// TwinCAT 3 PLC project Plc01_TrafficLightSystem
// ProgramVersion: 3.1.4020.4
// libraries:
//   Tc2_Standard, * (Beckhoff Automation GmbH)
//   Tc2_System, * (Beckhoff Automation GmbH)
//   Tc3_Module, * (Beckhoff Automation GmbH)
// project tree:
//   DUTs/Crossing/ E_CrossOpmodeState.TcDUT, E_CrossAutomaticState.TcDUT, E_CrossAutomaticActiveState.TcDUT, ST_CrossHmiData.TcDUT
//   DUTs/TrafficLight/ E_STLAutomaticActiveState.TcDUT, E_STLOpmodeState.TcDUT, E_STLAutomaticState.TcDUT, ST_STLHmiData.TcDUT
//   / PlcTask.TcTTO
//   POUs/Crossing/ FB_Crossing.TcPOU
//   POUs/Helpers/ FB_Blinker.TcPOU
//   POUs/ MAIN.TcPOU
//   POUs/TrafficLight/ FB_SingleTrafficLight.TcPOU
// real-time tasks:
//   TASK PlcTask: cycle T#10ms, priority 20, ADS port 350

CONFIGURATION Plc01_TrafficLightSystem
    RESOURCE PLC ON TwinCAT3
        TASK PlcTask(INTERVAL := T#10ms, PRIORITY := 20);
        PROGRAM MAIN WITH PlcTask : MAIN;
    END_RESOURCE
END_CONFIGURATION

// ---- DUTs/Crossing/E_CrossOpmodeState.TcDUT
//{attribute 'qualified_only'}
{attribute 'strict'}
TYPE E_CrossOpmodeState :
(
	eCrossOpmode_Commissioning 	:= 0,
	eCrossOpmode_Automatic 		:= 1
);
END_TYPE

// ---- DUTs/Crossing/E_CrossAutomaticState.TcDUT
//{attribute 'qualified_only'}
{attribute 'strict'}
TYPE E_CrossAutomaticState :
(
	eCrossAutomatic_StandBy := 0,
	eCrossAutomatic_Active 	:= 1	
);
END_TYPE

// ---- DUTs/Crossing/E_CrossAutomaticActiveState.TcDUT
//{attribute 'qualified_only'}
{attribute 'strict'}
TYPE E_CrossAutomaticActiveState :
(
	eCrossAutoActive_WaitBeforeH	:= 0,
	eCrossAutoActive_ReleaseH		:= 1,
	eCrossAutoActive_WaitBeforeV	:= 2,
	eCrossAutoActive_ReleaseV		:= 3 
);
END_TYPE

// ---- DUTs/Crossing/ST_CrossHmiData.TcDUT
TYPE ST_CrossHmiData :
STRUCT
	bInCommissioning			: BOOL;		// command signal commissioning mode (on rising edge)
	bInAutomatic				: BOOL;		// command signal automatic mode (on rising edge)
	bInAutomaticActive			: BOOL;		// command signal automatic active mode (on rising edge) -> traffic lights H1/2 and V1/2 alternate 
	bInAutomaticStandBy			: BOOL;		// command signal automatic stand by mode (on rising edge) -> on all traffic lights the yellow light blinks
	bOutCommissioningMode		: BOOL;		// status signal commissioning mode active
	bOutAutomaticMode			: BOOL;		// status signal automatic mode active
	sOutName					: STRING;	// crossing name
END_STRUCT
END_TYPE

// ---- DUTs/TrafficLight/E_STLAutomaticActiveState.TcDUT
//{attribute 'qualified_only'}
{attribute 'strict'}
TYPE E_STLAutomaticActiveState :
(
	eSTLAutoActive_Red 			:= 0,
	eSTLAutoActive_YellowRed	:= 1,
	eSTLAutoActive_Green 		:= 2,
	eSTLAutoActive_Yellow		:= 3 
);
END_TYPE

// ---- DUTs/TrafficLight/E_STLOpmodeState.TcDUT
//{attribute 'qualified_only'}
{attribute 'strict'}
TYPE E_STLOpmodeState :
(
	eSTLOpmode_Commissioning	:= 0,
	eSTLOpmode_Automatic 		:= 1
);
END_TYPE

// ---- DUTs/TrafficLight/E_STLAutomaticState.TcDUT
//{attribute 'qualified_only'}
{attribute 'strict'}
TYPE E_STLAutomaticState :
(
	eSTLAutomatic_StandBy 	:= 0,	
	eSTLAutomatic_Active 	:= 1
);
END_TYPE

// ---- DUTs/TrafficLight/ST_STLHmiData.TcDUT
TYPE ST_STLHmiData :
STRUCT
	bInCommissioning				: BOOL;		// command signal commissioning mode (on rising edge)
	bInCommissioningRedLightOn		: BOOL;		// test signal to toggle red light state (true/false -> on/off) 
	bInCommissioningYellowLightOn	: BOOL;		// test signal to toggle yellow light on (true/false -> on/off)
	bInCommissioningGreenLightOn	: BOOL;		// test signal to toggle green light on (true/false -> on/off)
	bInAutomatic					: BOOL;		// command signal automatic mode (on rising edge)
	bInAutomaticActive				: BOOL;		// command signal automatic active mode (on rising edge) -> red and green on request
	bInAutoActiveRedRequest			: BOOL;		// command signal request red (on rising edge)
	bInAutoActiveGreenRequest		: BOOL;		// command signal request green (on rising edge)
	bInAutomaticStandBy				: BOOL;		// command signal automatic stand by mode (on rising edge) -> yellow light blinks 
	bOutCommissioningMode			: BOOL;		// status signal commissioning mode active
	bOutAutomaticMode				: BOOL;		// status signal automatic mode active
	bOutAutomaticActiveMode			: BOOL;		// status signal automatic active mode active
	sOutName						: STRING;	// name of traffic light
	bOutRedLightStatus				: BOOL;		// status signal red light
	bOutYellowLightStatus			: BOOL;		// status signal yellow light
	bOutGreenLightStatus			: BOOL;		// status signal green light
END_STRUCT
END_TYPE

// ---- POUs/MAIN.TcPOU
PROGRAM MAIN
VAR
	// crossing with 4 traffic lights
	fbCrossing 		: FB_Crossing;
	// single traffic light
	fbTrafficLight 	: FB_SingleTrafficLight := (sInName := 'Traffic Light Single');
END_VAR

fbCrossing.M_Cycle();

fbTrafficLight.M_Cycle();

END_PROGRAM

// ---- POUs/Crossing/FB_Crossing.TcPOU
// Crossing with 4 TrafficLights
(*
			|		|
		  TL|		|
		  V2|		|TLH2
------------ --	 	 -------------
					|			
			|
------------	  -- -------------
		TLH1|		|TL
			|		|V1
			|		|
*)
FUNCTION_BLOCK FB_Crossing
VAR_INPUT
	// name
	sInName						: STRING; 	// name of crossing
	
	// commissioning mode
	bInCommissioning			: BOOL; 	// sensor signal commissioning mode (on rising edge)
	
	// automatic mode
	bInAutomatic				: BOOL; 	// sensor signal automatic mode (on rising edge)
	
	// automatic Active
	bInAutomaticActive			: BOOL; 	// sensor signal automatic active mode (on rising edge) -> traffic lights H1/2 and V1/2 alternate 
	
	// automatic stand by
	bInAutomaticStandBy			: BOOL;		// sensor signal automatic stand by mode (on rising edge) -> on all traffic lights the yellow light blinks  
	
END_VAR
VAR_OUTPUT
	// commissioning mode
	bOutCommissioningMode		: BOOL;		// status signal commissioning mode active
	
	// automatic mode
	bOutAutomaticMode			: BOOL;		// status signal automatic mode active

	// traffic lights
	fbTrafficLightH1	: FB_SingleTrafficLight;	// traffic light horizontal 1 (TLH1)
	fbTrafficLightH2	: FB_SingleTrafficLight;	// traffic light horizontal 2 (TLH2)
	fbTrafficLightV1	: FB_SingleTrafficLight;	// traffic light vertical 1 (TLV1)
	fbTrafficLightV2	: FB_SingleTrafficLight;	// traffic light vertical 2 (TLV2)
END_VAR
VAR
	// commissioning mode
	eOpmodeState				: E_CrossOpmodeState;			// opmode state
	fbRTrigInCommissioning		: R_TRIG;						// rising edge detection
	
	// automatic mode
	eAutomaticState				: E_CrossAutomaticState;		// automatic state
	fbRTrigInAutomatic			: R_TRIG;						// rising edge detection
	
	// automatic active
	eAutomaticActiveState		: E_CrossAutomaticActiveState;	// automatic active state
	fbRTrigInAutomaticActive	: R_TRIG;						// rising edge detection
	fbTimerReleaseH				: TON;							// timer horizontal traffic
	fbTimerWaitBeforeV			: TON;							// timer for waiting before releasing vertical traffic 
	fbTimerReleaseV				: TON;							// timer vertical traffic 
	fbTimerWaitBeforeH			: TON;							// timer for waiting before releasing horizontal traffic 
	
	// automatic stand by
	fbRTrigInAutomaticStandBy	: R_TRIG;						// rising edge detection
	
	// HMI data
	stHmiData					:ST_CrossHmiData;				// hmi data to interaction with hmi
	
END_VAR

METHOD FB_init : BOOL
VAR_INPUT
	bInitRetains : BOOL; // if TRUE, the retain variables are initialized (warm start / cold start)
	bInCopyCode : BOOL;  // if TRUE, the instance afterwards gets moved into the copy code (online change)
END_VAR
sInName := 'Crossing';
fbTrafficLightH1.sInName :=  'TL Horizontal 1';
fbTrafficLightH2.sInName :=  'TL Horizontal 2';
fbTrafficLightV1.sInName :=  'TL Vertical 1';
fbTrafficLightV2.sInName :=  'TL Vertical 2';
END_METHOD

METHOD M_AutoActiveHTGreenRequest : BOOL
VAR_INPUT
END_VAR
// horizontal traffic green request
fbTrafficLightH1.bInRedRequest 		:= FALSE;
fbTrafficLightH1.bInGreenRequest 	:= TRUE;
fbTrafficLightH2.bInRedRequest 		:= FALSE;
fbTrafficLightH2.bInGreenRequest 	:= TRUE;
			
fbTrafficLightV1.bInRedRequest 		:= FALSE;
fbTrafficLightV1.bInGreenRequest	:= FALSE;
fbTrafficLightV2.bInRedRequest 		:= FALSE;
fbTrafficLightV2.bInGreenRequest	:= FALSE;
END_METHOD

METHOD M_AutoActiveHTRedRequest : BOOL
VAR_INPUT
END_VAR
// horizontal traffic red request
fbTrafficLightH1.bInRedRequest		:= TRUE;
fbTrafficLightH1.bInGreenRequest 	:= FALSE;
fbTrafficLightH2.bInRedRequest 		:= TRUE;
fbTrafficLightH2.bInGreenRequest 	:= FALSE;
			
fbTrafficLightV1.bInRedRequest 		:= FALSE;
fbTrafficLightV1.bInGreenRequest 	:= FALSE;
fbTrafficLightV2.bInRedRequest 		:= FALSE;
fbTrafficLightV2.bInGreenRequest 	:= FALSE;
END_METHOD

METHOD M_AutoActiveVTGreenRequest : BOOL
VAR_INPUT
END_VAR
// vertical traffic green request
fbTrafficLightV1.bInRedRequest 		:= FALSE;
fbTrafficLightV1.bInGreenRequest 	:= TRUE;
fbTrafficLightV2.bInRedRequest 		:= FALSE;
fbTrafficLightV2.bInGreenRequest 	:= TRUE;
			
fbTrafficLightH1.bInRedRequest 		:= FALSE;
fbTrafficLightH1.bInGreenRequest	:= FALSE;
fbTrafficLightH2.bInRedRequest 		:= FALSE;
fbTrafficLightH2.bInGreenRequest	:= FALSE;
END_METHOD

METHOD M_AutoActiveVTRedRequest : BOOL
VAR_INPUT
END_VAR
// vertical traffic red request
fbTrafficLightV1.bInRedRequest		:= TRUE;
fbTrafficLightV1.bInGreenRequest 	:= FALSE;
fbTrafficLightV2.bInRedRequest 		:= TRUE;
fbTrafficLightV2.bInGreenRequest 	:= FALSE;
			
fbTrafficLightH1.bInRedRequest 		:= FALSE;
fbTrafficLightH1.bInGreenRequest 	:= FALSE;
fbTrafficLightH2.bInRedRequest 		:= FALSE;
fbTrafficLightH2.bInGreenRequest 	:= FALSE;
END_METHOD

METHOD M_Automatic : BOOL
VAR_INPUT
END_VAR
// automatic state machine
CASE eAutomaticState OF

	eCrossAutomatic_StandBy:
		M_AutomaticStandBy();
		IF fbRTrigInAutomaticActive.Q AND NOT fbRTrigInAutomaticStandBy.Q  THEN
			//IF M_SetAutomaticActiveModeTrafficLights() THEN
				eAutomaticActiveState := eCrossAutoActive_WaitBeforeH;
				eAutomaticState := eCrossAutomatic_Active;
			//END_IF
		END_IF

	eCrossAutomatic_Active:
		M_AutomaticActive();
		IF NOT fbRTrigInAutomaticActive.Q  AND fbRTrigInAutomaticStandBy.Q THEN
			//IF M_SetAutomaticStandByModeTrafficLights() THEN
				eAutomaticState := eCrossAutomatic_StandBy;
			//END_IF			
		END_IF
		
END_CASE
END_METHOD

METHOD M_AutomaticActive : BOOL
VAR_INPUT
END_VAR
// automatic active mode state machine
CASE eAutomaticActiveState OF
	
	// horizontal traffic will be released if vertical traffic stops
	eCrossAutoActive_WaitBeforeH:
		fbTimerReleaseH(PT:=T#2S);
		
		IF fbTrafficLightV1.bOutRedRequestReady AND fbTrafficLightV2.bOutRedRequestReady THEN
			fbTimerReleaseH.IN := TRUE;
		END_IF
		
		IF fbTimerReleaseH.Q THEN
			fbTimerReleaseH(IN:=FALSE);
			eAutomaticActiveState := eCrossAutoActive_ReleaseH;
		END_IF
	
	// horizontal traffic is released	
	eCrossAutoActive_ReleaseH:
		fbTimerWaitBeforeV(PT:=T#2S);
		
		IF fbTrafficLightH1.bOutGreenRequestReady AND fbTrafficLightH2.bOutGreenRequestReady THEN
			fbTimerWaitBeforeV.IN := TRUE;
		END_IF	
	
		IF fbTimerWaitBeforeV.Q THEN
			fbTimerWaitBeforeV(IN:=FALSE);
			eAutomaticActiveState := eCrossAutoActive_WaitBeforeV;
		END_IF
	
	// vertical traffic will be released if horizontal traffic stops
	eCrossAutoActive_WaitBeforeV:
		fbTimerReleaseV(PT:=T#2S);
		
		IF fbTrafficLightH1.bOutRedRequestReady AND fbTrafficLightH2.bOutRedRequestReady THEN
			fbTimerReleaseV.IN := TRUE;
		END_IF
		
		IF fbTimerReleaseV.Q THEN
			fbTimerReleaseV(IN:=FALSE);
			eAutomaticActiveState := eCrossAutoActive_ReleaseV;
		END_IF
	
	// vertical traffc is released	
	eCrossAutoActive_ReleaseV:
		fbTimerWaitBeforeH(PT:=T#2S);
		
		IF fbTrafficLightV1.bOutGreenRequestReady AND fbTrafficLightV2.bOutGreenRequestReady THEN
			fbTimerWaitBeforeH.IN := TRUE;
		END_IF	
		
		IF fbTimerWaitBeforeH.Q THEN
			fbTimerWaitBeforeH(IN:=FALSE);
			eAutomaticActiveState := eCrossAutoActive_WaitBeforeH;
		END_IF
	
END_CASE
END_METHOD

METHOD M_AutomaticStandBy : BOOL
VAR_INPUT
END_VAR
// reset timers
fbTimerReleaseH(IN:=FALSE);
fbTimerWaitBeforeV(IN:=FALSE);
fbTimerReleaseV(IN:=FALSE);
fbTimerWaitBeforeH(IN:=FALSE);
// implement additional functions for automatic stand by mode
END_METHOD

METHOD M_Commissioning : BOOL
VAR_INPUT
END_VAR
// implement additional functions for commissioning mode
END_METHOD

METHOD M_Cycle : BOOL
VAR_INPUT
END_VAR
// process input signals
M_Input();

// opmode state machine
CASE eOpmodeState OF
	
	eCrossOpmode_Commissioning:
		M_Commissioning();
		IF fbRTrigInAutomatic.Q AND NOT fbRTrigInCommissioning.Q THEN
			//IF M_SetAutomaticStandByModeTrafficLights() THEN
				eAutomaticState := eCrossAutomatic_StandBy;
				eOpmodeState := eCrossOpmode_Automatic;
			//END_IF
		END_IF
		
	eCrossOpmode_Automatic:
		M_Automatic();
		IF NOT fbRTrigInAutomatic.Q AND fbRTrigInCommissioning.Q THEN
			//IF M_SetCommissioningModeTrafficLights() THEN
				eOpmodeState := eCrossOpmode_Commissioning;
			//END_IF		
		END_IF

END_CASE

// set output signals
M_Output();
END_METHOD

METHOD M_Input : BOOL
VAR_INPUT
END_VAR
// process input signals

// commissioning mode
fbRTrigInCommissioning(CLK := bInCommissioning OR stHmiData.bInCommissioning);

// automatic mode
fbRTrigInAutomatic(CLK := bInAutomatic OR stHmiData.bInAutomatic);

// automatic Active
fbRTrigInAutomaticActive(CLK := bInAutomaticActive OR stHmiData.bInAutomaticActive);

// automatic stand by
fbRTrigInAutomaticStandBy(CLK := bInAutomaticStandBy OR stHmiData.bInAutomaticStandBy);
END_METHOD

METHOD M_Output : BOOL
VAR_INPUT
END_VAR
// set output signals

// execute traffic lights
fbTrafficLightH1.M_Cycle();
fbTrafficLightH2.M_Cycle();
fbTrafficLightV1.M_Cycle();
fbTrafficLightV2.M_Cycle();

IF eOpmodeState = eCrossOpmode_Automatic THEN
	// automatic mode
	bOutCommissioningMode := FALSE;
	bOutAutomaticMode := TRUE;
	M_SetAutomaticModeTrafficLights();
		
	IF eAutomaticState = eCrossAutomatic_Active THEN
		// automatic active mode
		M_SetAutomaticActiveModeTrafficLights();
			
		IF eAutomaticActiveState = eCrossAutoActive_WaitBeforeH THEN
			// vertical traffic red request
			M_AutoActiveVTRedRequest();
			
		ELSIF eAutomaticActiveState = eCrossAutoActive_ReleaseH THEN
			// horizontal traffic green request
			M_AutoActiveHTGreenRequest();
			
		ELSIF eAutomaticActiveState = eCrossAutoActive_WaitBeforeV THEN
			// horizontal traffic red request
			M_AutoActiveHTRedRequest();
			
		ELSIF eAutomaticActiveState = eCrossAutoActive_ReleaseV THEN
			// vertical traffic green request
			M_AutoActiveVTGreenRequest();
		END_IF
		
	ELSIF eAutomaticState = eCrossAutomatic_StandBy THEN
		// automatic stand by mode
		M_SetAutomaticStandByModeTrafficLights();
	ELSE
		// automatic stand by mode
		M_SetAutomaticStandByModeTrafficLights();
					
	END_IF

	
ELSIF eOpmodeState = eCrossOpmode_Commissioning THEN
	// commissioning mode
	bOutCommissioningMode := TRUE;
	bOutAutomaticMode := FALSE;
	M_SetCommissioningModeTrafficLights();
	
ELSE
	// commissioning mode
	bOutCommissioningMode := TRUE;
	bOutAutomaticMode := FALSE;
	M_SetCommissioningModeTrafficLights();
	
END_IF

// hmi output data
stHmiData.sOutName := sInName;
stHmiData.bOutCommissioningMode := bOutCommissioningMode;
stHmiData.bOutAutomaticMode := bOutAutomaticMode;
END_METHOD

METHOD M_SetAutomaticActiveModeTrafficLights : BOOL
VAR_INPUT
END_VAR
// set all traffic lights to automatic active mode
fbTrafficLightH1.bInAutomaticStandBy := FALSE;
fbTrafficLightH2.bInAutomaticStandBy := FALSE;
fbTrafficLightV1.bInAutomaticStandBy := FALSE;
fbTrafficLightV2.bInAutomaticStandBy := FALSE;

fbTrafficLightH1.bInAutomaticActive := TRUE;
fbTrafficLightH2.bInAutomaticActive := TRUE;
fbTrafficLightV1.bInAutomaticActive := TRUE;
fbTrafficLightV2.bInAutomaticActive := TRUE;

fbTrafficLightV1.bInRedRequest 			:= FALSE;
fbTrafficLightV1.bInGreenRequest 		:= FALSE;
fbTrafficLightV2.bInRedRequest 			:= FALSE;
fbTrafficLightV2.bInGreenRequest 		:= FALSE;	

fbTrafficLightH1.bInRedRequest 			:= FALSE;
fbTrafficLightH1.bInGreenRequest 		:= FALSE;
fbTrafficLightH2.bInRedRequest 			:= FALSE;
fbTrafficLightH2.bInGreenRequest 		:= FALSE;

M_SetAutomaticActiveModeTrafficLights := TRUE;
END_METHOD

METHOD M_SetAutomaticModeTrafficLights : BOOL
VAR_INPUT
END_VAR
// set all traffic lights to automatic mode

// vertical traffic automatic mode
fbTrafficLightV1.bInCommissioning 	:= FALSE;
fbTrafficLightV2.bInCommissioning 	:= FALSE;
fbTrafficLightV1.bInAutomatic 		:= TRUE;
fbTrafficLightV2.bInAutomatic 		:= TRUE;
// horizontal traffic automatic mode
fbTrafficLightH1.bInCommissioning 	:= FALSE;
fbTrafficLightH2.bInCommissioning 	:= FALSE;
fbTrafficLightH1.bInAutomatic 		:= TRUE;
fbTrafficLightH2.bInAutomatic 		:= TRUE;

M_SetAutomaticModeTrafficLights := TRUE;
END_METHOD

METHOD M_SetAutomaticStandByModeTrafficLights : BOOL
VAR_INPUT
END_VAR
// set all traffic lights to automatic stand by mode

fbTrafficLightH1.bInAutomaticActive := FALSE;
fbTrafficLightH2.bInAutomaticActive := FALSE;
fbTrafficLightV1.bInAutomaticActive := FALSE;
fbTrafficLightV2.bInAutomaticActive := FALSE;

fbTrafficLightH1.bInAutomaticStandBy := TRUE;
fbTrafficLightH2.bInAutomaticStandBy := TRUE;
fbTrafficLightV1.bInAutomaticStandBy := TRUE;
fbTrafficLightV2.bInAutomaticStandBy := TRUE;

// reset request signals
fbTrafficLightV1.bInRedRequest 			:= FALSE;
fbTrafficLightV1.bInGreenRequest 		:= FALSE;
fbTrafficLightV2.bInRedRequest 			:= FALSE;
fbTrafficLightV2.bInGreenRequest 		:= FALSE;		
	
fbTrafficLightH1.bInRedRequest 			:= FALSE;
fbTrafficLightH1.bInGreenRequest 		:= FALSE;
fbTrafficLightH2.bInRedRequest 			:= FALSE;
fbTrafficLightH2.bInGreenRequest 		:= FALSE;

M_SetAutomaticStandByModeTrafficLights := TRUE;
END_METHOD

METHOD M_SetCommissioningModeTrafficLights : BOOL
VAR_INPUT
END_VAR
// set all traffic lights to commissioning mode

fbTrafficLightH1.bInAutomatic := FALSE;
fbTrafficLightH2.bInAutomatic := FALSE;
fbTrafficLightV1.bInAutomatic := FALSE;
fbTrafficLightV2.bInAutomatic := FALSE;

fbTrafficLightH1.bInAutomaticActive := FALSE;
fbTrafficLightH2.bInAutomaticActive := FALSE;
fbTrafficLightV1.bInAutomaticActive := FALSE;
fbTrafficLightV2.bInAutomaticActive := FALSE;

fbTrafficLightH1.bInAutomaticStandBy := TRUE;
fbTrafficLightH2.bInAutomaticStandBy := TRUE;
fbTrafficLightV1.bInAutomaticStandBy := TRUE;
fbTrafficLightV2.bInAutomaticStandBy := TRUE;

fbTrafficLightH1.bInCommissioning := TRUE;
fbTrafficLightH2.bInCommissioning := TRUE;
fbTrafficLightV1.bInCommissioning := TRUE;
fbTrafficLightV2.bInCommissioning := TRUE;

M_SetCommissioningModeTrafficLights := TRUE;
END_METHOD

END_FUNCTION_BLOCK

// ---- POUs/TrafficLight/FB_SingleTrafficLight.TcPOU
// single traffic light

(*
	 _
	| |
	|o| red light
	|o| yellow light
	|o| green light
	|_|
	
*)

FUNCTION_BLOCK FB_SingleTrafficLight
VAR_INPUT
	// name
	sInName						: STRING; 	// name of traffic light
	
	// commissioning mode
	bInCommissioning			: BOOL; 	// sensor signal commissioning mode (on rising edge)
	bInRedLightOn				: BOOL;		// test signal to toggle red light state (true/false -> on/off) 
	bInYellowLightOn			: BOOL;		// test signal to toggle yellow light on (true/false -> on/off)
	bInGreenLightOn				: BOOL;		// test signal to toggle green light on (true/false -> on/off)
		
	// automatic mode
	bInAutomatic				: BOOL; 	// sensor signal automatic mode (on rising edge)
	
	// automatic active
	bInAutomaticActive			: BOOL; 	// sensor signal automatic active mode (on rising edge) -> red and green on request

	bInRedRequest				: BOOL;		// sensor signal request red (on rising edge)
	bInGreenRequest				: BOOL;		// sensor signal request green (on rising edge)
	
	// automatic stand by
	bInAutomaticStandBy			: BOOL;		// sensor signal automatic stand by mode (on rising edge) -> yellow light blinks  
	
END_VAR
VAR_OUTPUT
	// lights
	bOutRedLight		AT %Q* 	: BOOL;  	// actor signal red light
	bOutYellowLight		AT %Q* 	: BOOL; 	// actor signal yellow light
	bOutGreenLight		AT %Q* 	: BOOL; 	// actor signal green light
	
	// commissioning mode
	bOutCommissioningMode		: BOOL;		// status signal commissioning mode active
	
	// automatic mode
	bOutAutomaticMode			: BOOL;		// status signal automatic mode active
	bOutAutomaticActiveMode		: BOOL;		// status signal automatic active mode active
	
	// automatic active
	bOutRedRequestReady			: BOOL;		// signal red state reached
	bOutGreenRequestReady		: BOOL;		// signal green state reached
	
END_VAR
VAR
	// commissioning mode
	eOpmodeState				: E_STLOpmodeState;				// opmode state
	fbRTrigInCommissioning		: R_TRIG;						// rising edge detection
	
	// automatic mode
	eAutomaticState				: E_STLAutomaticState;			// automatic state
	fbRTrigInAutomatic			: R_TRIG;						// rising edge detection
	
	// automatic active
	eAutomaticActiveState		: E_STLAutomaticActiveState;	// automatic state
	fbRTrigInAutomaticActive	: R_TRIG;						// rising edge detection
	fbTimerRed					: TON;							// timer for activate red state
	fbTimerYellowRed			: TON;							// timer for activate yellow red state
	fbTimerGreen				: TON;							// timer for activate green state
	fbTimerYellow				: TON;							// timer for activate yellow state
	fbRTrigInRedRequest			: R_TRIG;						// rising edge detection
	fbRTrigInGreenRequest		: R_TRIG;						// rising edge detection 
	
	// automatic stand by
	fbRTrigInAutomaticStandBy	: R_TRIG;						// rising edge detection 
	fbBlinker					: FB_Blinker;					// blinker
	
	// HMI Data
	stHmiData					: ST_STLHmiData;				// hmi data to interaction with hmi
	
END_VAR

METHOD M_Automatic : BOOL
VAR_INPUT
END_VAR
// automatic state machine
CASE eAutomaticState OF

	eSTLAutomatic_StandBy:
		M_AutomaticStandBy();
		IF fbRTrigInAutomaticActive.Q AND NOT fbRTrigInAutomaticStandBy.Q  THEN
			bOutRedRequestReady := FALSE;
			bOutGreenRequestReady := FALSE;
			eAutomaticActiveState := eSTLAutoActive_Red;
			eAutomaticState := eSTLAutomatic_Active;
		END_IF

	eSTLAutomatic_Active:
		M_AutomaticActive();
		IF NOT fbRTrigInAutomaticActive.Q  AND fbRTrigInAutomaticStandBy.Q THEN
			eAutomaticState := eSTLAutomatic_StandBy;			
		END_IF
		
END_CASE
END_METHOD

METHOD M_AutomaticActive : BOOL
VAR_INPUT
END_VAR
// automatic active mode state machine
CASE eAutomaticActiveState OF
	
	// red state and waiting on green request
	eSTLAutoActive_Red:
		bOutRedRequestReady := TRUE;
		bOutGreenRequestReady := FALSE;
	
		fbTimerYellowRed(PT:=T#2S);
		IF fbRTrigInGreenRequest.Q THEN
			fbTimerYellowRed.IN := TRUE;
		END_IF
		IF fbTimerYellowRed.Q THEN
			fbTimerYellowRed(IN:=FALSE);
			eAutomaticActiveState := eSTLAutoActive_YellowRed;
		END_IF
	
	// yellow red state	
	eSTLAutoActive_YellowRed:
		bOutRedRequestReady := FALSE;
		bOutGreenRequestReady := FALSE;
		
		fbTimerGreen(IN:=TRUE,PT:=T#2S);
		IF fbTimerGreen.Q THEN
			fbTimerGreen(IN:=FALSE);
			eAutomaticActiveState := eSTLAutoActive_Green;
		END_IF

	// green state and waiting on red request
	eSTLAutoActive_Green:
		bOutRedRequestReady := FALSE;
		bOutGreenRequestReady := TRUE;	
		
		fbTimerYellow(PT:=T#2S);
		IF fbRTrigInRedRequest.Q THEN
			fbTimerYellow.IN := TRUE;
		END_IF
		IF fbTimerYellow.Q THEN
			fbTimerYellow(IN:=FALSE);
			eAutomaticActiveState := eSTLAutoActive_Yellow;
		END_IF
	
	// yellow state	
	eSTLAutoActive_Yellow:
		bOutRedRequestReady := FALSE;
		bOutGreenRequestReady := FALSE;
		
		fbTimerRed(IN:=TRUE,PT:=T#2S);
		IF fbTimerRed.Q THEN
			fbTimerRed(IN:=FALSE);
			eAutomaticActiveState := eSTLAutoActive_Red;
		END_IF
	
END_CASE
END_METHOD

METHOD M_AutomaticStandBy : BOOL
VAR_INPUT
END_VAR
// reset timers
fbTimerYellowRed(IN:=FALSE);
fbTimerGreen(IN:=FALSE);
fbTimerYellow(IN:=FALSE);
fbTimerRed(IN:=FALSE);
// implement additional functions for automatic stand by mode
END_METHOD

METHOD M_Commissioning : BOOL
VAR_INPUT
END_VAR
// implement additional functions for commissioning mode
END_METHOD

METHOD M_Cycle : BOOL
VAR_INPUT
END_VAR
// process input signals
M_Input();

// opmode state machine
CASE eOpmodeState OF
	
	eSTLOpmode_Commissioning:
		M_Commissioning();
		IF fbRTrigInAutomatic.Q AND NOT fbRTrigInCommissioning.Q THEN
			eAutomaticState := eSTLAutomatic_StandBy;	
			eOpmodeState := eSTLOpmode_Automatic;
		END_IF
		
	eSTLOpmode_Automatic:
		M_Automatic();
		IF NOT fbRTrigInAutomatic.Q AND fbRTrigInCommissioning.Q THEN
			eOpmodeState := eSTLOpmode_Commissioning;
		END_IF

END_CASE

// set output signals
M_Output();
END_METHOD

METHOD M_Input : BOOL
VAR_INPUT
END_VAR
// process input signals

// commissioning mode
fbRTrigInCommissioning(CLK := bInCommissioning OR stHmiData.bInCommissioning);

// automatic mode
fbRTrigInAutomatic(CLK := bInAutomatic OR stHmiData.bInAutomatic);

// automatic Active
fbRTrigInAutomaticActive(CLK := bInAutomaticActive OR stHmiData.bInAutomaticActive);


fbRTrigInRedRequest(CLK := bInRedRequest OR stHmiData.bInAutoActiveRedRequest);
fbRTrigInGreenRequest(CLK := bInGreenRequest OR stHmiData.bInAutoActiveGreenRequest);

// automatic stand by
fbRTrigInAutomaticStandBy(CLK := bInAutomaticStandBy OR stHmiData.bInAutomaticStandBy);
END_METHOD

METHOD M_Output : BOOL
VAR_INPUT
END_VAR
// set output signals

// commissioning mode
IF (eOpmodeState = eSTLOpmode_Commissioning) THEN
	bOutCommissioningMode := TRUE;
ELSE
	bOutCommissioningMode := FALSE;
END_IF

// automatic mode
IF (eOpmodeState = eSTLOpmode_Automatic) THEN
	bOutAutomaticMode := TRUE;
ELSE
	bOutAutomaticMode := FALSE;
END_IF

IF (eAutomaticState = eSTLAutomatic_Active) THEN
	bOutAutomaticActiveMode := TRUE;
ELSE
	bOutAutomaticActiveMode := FALSE;	
END_IF

// red light
IF (eOpmodeState = eSTLOpmode_Automatic AND eAutomaticState = eSTLAutomatic_Active) AND (eAutomaticActiveState = eSTLAutoActive_Red OR eAutomaticActiveState = eSTLAutoActive_YellowRed) 
	OR eOpmodeState = eSTLOpmode_Commissioning AND (bInRedLightOn OR stHmiData.bInCommissioningRedLightOn) THEN
	bOutRedLight := TRUE;
ELSE
	bOutRedLight := FALSE;
END_IF

// yellow light
IF (eOpmodeState = eSTLOpmode_Automatic AND eAutomaticState = eSTLAutomatic_Active)  AND (eAutomaticActiveState = eSTLAutoActive_Yellow OR eAutomaticActiveState = eSTLAutoActive_YellowRed) 
	OR eOpmodeState = eSTLOpmode_Commissioning AND (bInYellowLightOn OR stHmiData.bInCommissioningYellowLightOn) THEN
	fbBlinker(CLK := FALSE);
	bOutYellowLight := TRUE;
ELSIF  eOpmodeState = eSTLOpmode_Automatic AND eAutomaticState = eSTLAutomatic_StandBy THEN
	fbBlinker(CLK := TRUE);
	bOutYellowLight := fbBlinker.Q;
ELSE
	fbBlinker(CLK := FALSE);
	bOutYellowLight := FALSE;
END_IF

// green light
IF (eOpmodeState = eSTLOpmode_Automatic AND eAutomaticState = eSTLAutomatic_Active) AND (eAutomaticActiveState = eSTLAutoActive_Green) 
	OR eOpmodeState = eSTLOpmode_Commissioning AND (bInGreenLightOn OR stHmiData.bInCommissioningGreenLightOn) THEN
	bOutGreenLight := TRUE;
ELSE
	bOutGreenLight := FALSE;
END_IF

// hmi output data
stHmiData.sOutName := sInName;
stHmiData.bOutCommissioningMode := bOutCommissioningMode;
stHmiData.bOutAutomaticMode := bOutAutomaticMode;
stHmiData.bOutAutomaticActiveMode := bOutAutomaticActiveMode;
stHmiData.bOutRedLightStatus := bOutRedLight;
stHmiData.bOutYellowLightStatus := bOutYellowLight;
stHmiData.bOutGreenLightStatus := bOutGreenLight;
END_METHOD

END_FUNCTION_BLOCK

// ---- POUs/Helpers/FB_Blinker.TcPOU
FUNCTION_BLOCK FB_Blinker
VAR_INPUT
	CLK: BOOL;
END_VAR
VAR_OUTPUT
	Q: BOOL;
END_VAR
VAR
	fbTimer1: TON;
	fbTimer2: TON;
END_VAR

fbTimer1(IN :=(NOT fbTimer2.Q AND CLK), PT := T#1S);
fbTimer2(IN := fbTimer1.Q, PT := T#1S);
Q := fbTimer1.Q;

END_FUNCTION_BLOCK
